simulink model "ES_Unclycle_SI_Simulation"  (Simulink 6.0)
settings: Solver=ode45  StartTime=0.0  StopTime=tmax  FixedStep=deltaT  MaxStep=deltaT+.001  MinStep=deltaT-.001  RelTol=1e-3
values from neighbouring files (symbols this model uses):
  ax = .05    (= 0.05)    [ES_Unicycle_Values_SI.m]    (also in ES_PointMass_Values.m; ES_SimplifyPointMass_Values.m; ES_Unstable_Values.m; doublepointmass.m)
  ay = .05    (= 0.05)    [ES_Unicycle_Values_SI.m]    (also in ES_PointMass_Values.m; ES_SimplifyPointMass_Values.m; ES_Unstable_Values.m; doublepointmass.m)
  centx = 0    [ES_Unicycle_nc_values_tune_V.m]    (also in ES_Unicycle_nc_values_tune_V_moving.m; ES_Unicycle_Values.m; ES_Unicycle_Values_SI.m = -1; ES_PointMass_Values.m = -1)
  centy = 0    [ES_Unicycle_nc_values_tune_V.m]    (also in ES_Unicycle_nc_values_tune_V_moving.m; ES_Unicycle_Values.m; ES_Unicycle_Values_SI.m = -1; ES_PointMass_Values.m = -1)
  cx = 20    [ES_Unicycle_Values.m]    (also in ES_Unicycle_Values_SI.m = 10; ES_PointMass_Values.m; ES_SimplifyPointMass_Values.m = 15; ES_Unstable_Values.m = 15)
  cy = 20    [ES_Unicycle_Values.m]    (also in ES_Unicycle_Values_SI.m = 10; ES_PointMass_Values.m; ES_SimplifyPointMass_Values.m = 15; ES_Unstable_Values.m = 15)
  ICx = 2 - r    (= 1.8)    [ES_Unicycle_nc_values_tune_V.m]    (also in ES_Unicycle_nc_values_tune_V_moving.m = 1.5; ES_Unicycle_Values.m = 2; ES_Unicycle_Values_SI.m = 1; ES_PointMass_Values.m = 1)
  ICy = 2    [ES_Unicycle_nc_values_tune_V.m]    (also in ES_Unicycle_nc_values_tune_V_moving.m; ES_Unicycle_Values.m = 1; ES_Unicycle_Values_SI.m = 1; ES_PointMass_Values.m = 1)
  p1 = 1    [ES_Unicycle_Values_SI.m]    (also in doublepointmass.m; pointmass.m)
  p2 = 1/2    (= 0.5)    [ES_Unicycle_Values_SI.m]    (also in doublepointmass.m; pointmass.m)
  root = 1    [ES_Unicycle_Values_SI.m]    (also in ES_PointMass_Values.m; ES_SimplifyPointMass_Values.m; ES_Unstable_Values.m; doublepointmass.m)
  tmax = 50    [ES_Unicycle_nc_values_tune_V.m]    (also in ES_Unicycle_nc_values_tune_V_moving.m = 300; ES_Unicycle_Values.m = 25; ES_Unicycle_Values_SI.m = 150; ES_PointMass_Values.m)
  wx = 20    [ES_Unicycle_Values_SI.m]    (also in ES_PointMass_Values.m = 30; ES_SimplifyPointMass_Values.m = 30; ES_Unstable_Values.m = 30; doublepointmass.m = 30)
  wy = 20    [ES_Unicycle_Values_SI.m]    (also in ES_PointMass_Values.m = 30; ES_SimplifyPointMass_Values.m = 30; ES_Unstable_Values.m = 30; doublepointmass.m = 30)
undefined symbols (not defined in the file or in its folder): Graph, sfunxy, simulink3, Sinks, XY
libraries: simulink x1

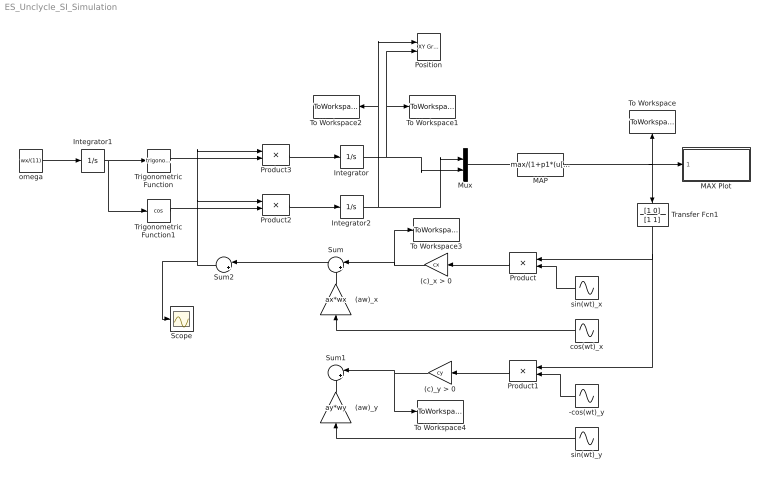
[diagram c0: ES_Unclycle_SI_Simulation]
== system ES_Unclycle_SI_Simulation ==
  (aw)_x : Gain  Orientation=up  Gain=ax*wx
  (aw)_y : Gain  Orientation=up  Gain=ay*wy
  (c)_x > 0 : Gain  Orientation=left  Gain=cx
  (c)_y > 0 : Gain  Orientation=left  Gain=cy
  -cos(wt)_y : Sin  Orientation=left  Amplitude=-1  Frequency=wy  Phase=pi/2  SampleTime=0
  Integrator : Integrator  InitialCondition=ICy
  Integrator1 : Integrator  InitialCondition=ICy
  Integrator2 : Integrator  InitialCondition=ICx
  MAP : Fcn  Expr=max/(1+p1*(u[1]-centx)^2+p2*(u[2]-centy)^2)^(root)
  MAX Plot : Subsystem
  Mux : Mux  Inputs=2
  Position : simulink/Sinks/XY Graph  xmin=centx - abs(ICx) -1  xmax=centx + abs(ICx) + 2  ymin=centy - abs(ICy)-1  ymax=centy + abs(ICy) + 2  st=-1
  Product : Product  Orientation=left
  Product1 : Product  Orientation=left
  Product2 : Product
  Product3 : Product
  Scope : Scope
  Sum : Sum  Orientation=left  Inputs=|++
  Sum1 : Sum  Orientation=left  Inputs=|++
  Sum2 : Sum  Orientation=left  Inputs=|++
  To Workspace : ToWorkspace  VariableName=MAX  SampleTime=-1  SaveFormat=Array
  To Workspace1 : ToWorkspace  VariableName=Y  SampleTime=-1  SaveFormat=Array
  To Workspace2 : ToWorkspace  VariableName=X  SampleTime=-1  SaveFormat=Array
  To Workspace3 : ToWorkspace  VariableName=Vx  SampleTime=-1  SaveFormat=Array
  To Workspace4 : ToWorkspace  VariableName=Vy  SampleTime=-1  SaveFormat=Array
  Transfer Fcn1 : TransferFcn  Orientation=down  Numerator=[1 0]  Denominator=[1 1]
  Trigonometric Function : Trigonometry
  Trigonometric Function1 : Trigonometry  Operator=cos
  cos(wt)_x : Sin  Orientation=left  Frequency=wx  Phase=pi/2  SampleTime=0
  omega : Constant  Value=wx/(11)
  sin(wt)_x : Sin  Orientation=left  Frequency=wx  SampleTime=0
  sin(wt)_y : Sin  Orientation=left  Frequency=wy  SampleTime=0
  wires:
  Integrator/1 -> To Workspace1/1, Position/2, Mux/2
  Integrator2/1 -> Mux/1, To Workspace2/1, Position/1
  (aw)_y/1 -> Sum1/2
  (aw)_x/1 -> Sum/2
  sin(wt)_x/1 -> Product/2
  (c)_y > 0/1 -> Sum1/1, To Workspace4/1
  (c)_x > 0/1 -> Sum/1, To Workspace3/1
  Product1/1 -> (c)_y > 0/1
  cos(wt)_x/1 -> (aw)_x/1
  Product/1 -> (c)_x > 0/1
  Mux/1 -> MAP/1
  MAP/1 -> MAX Plot/1(MAX Seeking Value), To Workspace/1, Transfer Fcn1/1
  -cos(wt)_y/1 -> Product1/2
  sin(wt)_y/1 -> (aw)_y/1
  Transfer Fcn1/1 -> Product/1, Product1/1
  omega/1 -> Integrator1/1
  Integrator1/1 -> Trigonometric Function/1, Trigonometric Function1/1
  Product3/1 -> Integrator/1
  Product2/1 -> Integrator2/1
  Trigonometric Function1/1 -> Product2/2
  Trigonometric Function/1 -> Product3/2
  Sum1/1 -> ?
  Sum/1 -> Sum2/1
  Sum2/1 -> Product3/1, Product2/1, Scope/1

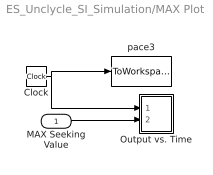
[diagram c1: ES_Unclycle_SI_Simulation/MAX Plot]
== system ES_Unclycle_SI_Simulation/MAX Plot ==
  MAX Seeking Value : Inport  Port=1  LatchInput=off
  Clock : Clock
  Output vs. Time : Subsystem  AncestorBlock=simulink3/Sinks/XY Graph  LoadFcn=sfunxy([],[],[],'LoadBlock')  StartFcn=sfunxy([],[],[],'Start')  StopFcn=sfunxy([],[],[],'Stop')  TreatAsAtomicUnit=on  SimViewingDevice=on  mask(XY scope.){xmin=0, xmax=tmax, ymin=-3, ymax=max + 2, st=-1}
      mask prompts: xmin "x-min:"; xmax "x-max:"; ymin "y-min:"; ymax "y-max:"; st "Sample time:"
      mask help: XY scope using MATLAB graph window. First input is used as time base. Enter plotting ranges.
  pace3 : ToWorkspace  VariableName=T  SampleTime=-1  SaveFormat=Array
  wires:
  Clock/1 -> pace3/1, Output vs. Time/1(time)
  MAX Seeking Value/1 -> Output vs. Time/2(MAX Seeking Value)

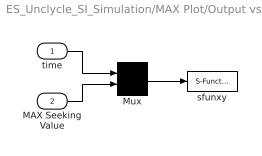
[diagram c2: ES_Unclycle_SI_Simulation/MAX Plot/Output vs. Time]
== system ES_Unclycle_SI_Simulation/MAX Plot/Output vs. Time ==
  time : Inport  Port=1  LatchInput=off
  MAX Seeking Value : Inport  Port=2  LatchInput=off
  Mux : Mux  Inputs=2
  sfunxy : S-Function  FunctionName=sfunxy  Parameters=[xmin xmax ymin ymax], st
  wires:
  Mux/1 -> sfunxy/1
  time/1 -> Mux/1
  MAX Seeking Value/1 -> Mux/2
